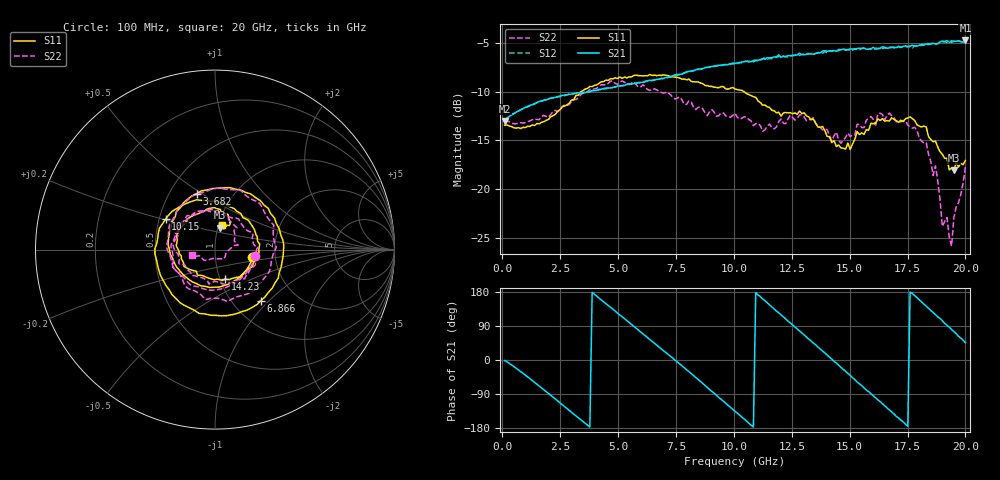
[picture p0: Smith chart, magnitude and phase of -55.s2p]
!Agilent Technologies,N5230C,MY49001569,A.09.33.09
!Agilent N5230C: A.09.33.09
!Date: Sunday, July 26, 2015 12:30:22
!Correction: S11(Full 2 Port(1,2))
!S21(Full 2 Port(1,2))
!S12(Full 2 Port(1,2))
!S22(Full 2 Port(1,2))
!S2P File: Measurements: S11, S21, S12, S22:
# Hz S  dB  R 50
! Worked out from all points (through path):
!   201 points, 100 MHz to 20 GHz, reference 50 ohm
!   highest |S21| = -4.76 dB at 20 GHz (marker M1); lowest = -13.0 dB at 100 MHz (marker M2)
!   group delay of S21, straight-line fit = 145 ps
!   lowest |S11| = -18.1 dB at 19.5 GHz (marker M3), VSWR 1.29, Z = 51.2 + j12.7 ohm
!   |S11| at or under -10 dB: start of sweep to 3.414 GHz; 10.43 GHz to end of sweep
!   |S22| runs from -25.9 to -8.9 dB; largest |S21 - S12| = 0.032
!   S11 on the Smith chart (normalised r, x): 100 MHz: 1.52, -0.12; 3.682 GHz: 0.68, +0.48; 6.866 GHz: 1.34, -0.89; 10.15 GHz: 0.54, +0.20; 14.23 GHz: 1.06, -0.36; 20 GHz: 1.04, +0.29
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1e8  -13.46 -10.4  -13.01 -1.5  -12.93 -1.2  -12.98 -8.5
1.692e9  -13.15 -125.9  -11.00 -73.3  -10.97 -73.3  -12.58 -120.4
3.483e9  -9.92 118.7  -10.09 -162.2  -10.14 -162.5  -10.16 129.6
3.682e9  -9.68 107.9  -10.03 -172.3  -10.02 -172.4  -10.00 118.1
5.473e9  -8.49 17.6  -9.20 99.0  -9.24 98.4  -9.30 30.9
6.7665e9  -8.33 -43.4  -8.73 34.3  -8.72 34.1  -9.97 -29.9
6.866e9  -8.36 -48.4  -8.65 29.5  -8.68 28.7  -10.08 -35.8
8.7565e9  -9.39 -139.0  -7.57 -67.1  -7.54 -68.0  -12.17 -137.5
1.005e10  -9.74 153.5  -7.11 -135.5  -7.16 -136.4  -12.23 143.1
1.01495e10  -9.81 148.5  -7.07 -140.3  -7.13 -141.4  -12.63 138.4
1.11445e10  -11.12 99.7  -6.71 167.3  -6.80 166.3  -13.50 79.5
1.204e10  -12.53 49.1  -6.50 118.8  -6.39 118.1  -12.82 21.7
1.3433e10  -12.81 -25.0  -6.17 44.8  -6.22 44.1  -12.68 -44.6
1.4229e10  -15.23 -71.4  -5.83 2.4  -5.89 1.6  -15.05 -89.2
1.5622e10  -14.39 -169.1  -5.55 -73.7  -5.54 -73.9  -13.70 -172.5
1.67165e10  -13.02 134.9  -5.52 -132.1  -5.41 -132.4  -12.21 129.2
1.801e10  -13.54 77.0  -5.24 158.9  -5.28 156.7  -14.79 64.9
1.87065e10  -15.07 61.1  -5.11 119.8  -5.16 118.8  -17.63 11.3
1.9005e10  -16.44 64.6  -4.83 103.5  -4.93 101.0  -23.82 -13.9
1.9403e10  -17.84 72.9  -4.94 80.5  -4.79 78.9  -25.85 -104.4
1.95025e10  -18.07 77.6  -4.85 75.2  -4.81 73.6  -22.90 -125.3
2e10  -17.07 74.3  -4.76 45.8  -4.78 44.4  -17.74 -166.1
